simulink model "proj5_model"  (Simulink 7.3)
settings: Solver=FixedStepDiscrete  StartTime=0.0  StopTime=1.2  RelTol=1e-3
InitFcn:
  | clear
  | % Digital Modulation
  | M=4;                % MQAM
  | Fs=1e06;             % Symbols Rate
  | Fb=log2(M)*Fs;   % bit rate
  | 
  | % Power Transmitted and Received
  | PT=5.0;             % Transmitted Power in Watts
  | A=1/100;           % channel attenuation
  | PR=A*PT;          % Received Power in Watts
  | 
  | % channel
  | P=[0,-5, 5];   % dB
  | T=[0, 10 15]*10^(-6);  % sec
  | fd=60; %Hz
libraries: commrandsrc2 x1, commsink2 x1, commchan3 x1, commdigbbndam3 x1

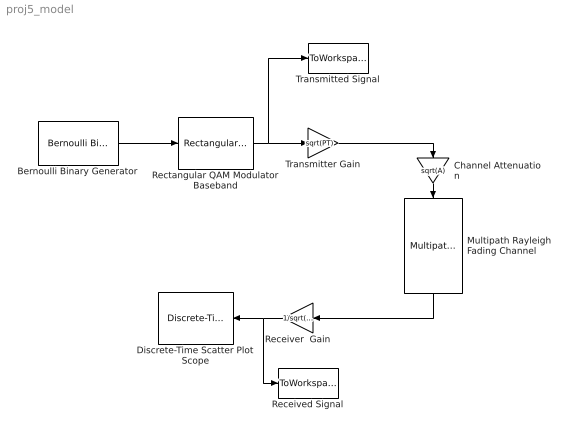
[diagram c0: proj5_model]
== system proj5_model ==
  Bernoulli Binary Generator : commrandsrc2/Bernoulli Binary Generator  DialogController=commDDGCreate  DialogControllerArgs=DataTag0  SystemSampleTime=-1  P=0.5  seed=61  Ts=1/Fb  frameBased=on  sampPerFrame=log2(M)*100  orient=off  outDataType=single
  Channel Attenuation : Gain  Gain=sqrt(A)  ParameterDataType=sfix(16)  ParameterScaling=2^0  OutDataType=sfix(16)  OutScaling=2^0
  Discrete-Time Scatter Plot Scope : commsink2/Discrete-Time Scatter Plot Scope  Tag=ScatterPlot  SystemSampleTime=-1  sampPerSymb=1  offsetEye=0  numTraces=40  numNewFrames=10  LineMarkers=.  LineColors=b  fading=on  render=on  AxisGrid=on  xMin=-3.3  xMax=3.315  yMin=-3.3  yMax=3.315  inphaseLabel=In-phase Amplitude  quadratureLabel=Quadrature Amplitude  openScopeAtSimStart=on  FrameNumber=off  FigPos=[232 106 560 560]  figTitle=Scatter Plot  numLinesMax=8  block_type_=scatter
  Multipath Rayleigh Fading Channel : commchan3/Multipath Rayleigh Fading Channel  SystemSampleTime=-1  maxDopplerShift=fd  spectrumType=Jakes  sigmaGaussian=1/sqrt(2)  coeffRounded=[1 -1.72 0.785]  freqMinMaxRJakes=[0 1]  freqMinMaxAJakes=[0 1]  sigmaGaussian1=1/sqrt(2)  sigmaGaussian2=1/sqrt(2)  centerFreqGaussian1=0.0  centerFreqGaussian2=0.0  gainGaussian1=0.5  gainGaussian2=0.5  coeffBell=9  dopplerSpectrum=doppler.jakes  pathDelays=T  avgPathGaindB=P  normalizePathGains=on  seed=73  enableProbe=0  openVisAtStart=off  outPathGains=off  outDelay=off
  Received Signal : ToWorkspace  VariableName=y  SampleTime=-1  SaveFormat=Array
  Receiver  Gain : Gain  Gain=1/sqrt(PR)  ParameterDataType=sfix(16)  ParameterScaling=2^0  OutDataType=sfix(16)  OutScaling=2^0
  Rectangular QAM Modulator Baseband : commdigbbndam3/Rectangular QAM Modulator Baseband  DialogController=commDDGCreate  DialogControllerArgs=DataTag1  M=M  InType=Bit  Enc=Gray  Mapping=[0:15]  PowType=Average Power  MinDist=2  AvgPow=1  PeakPow=1  Ph=0  outDtype=double  outWordLen=16  outUDDataType=sfix(16)  outFracLenMode=Best precision  outFracLen=15
  Transmitted Signal : ToWorkspace  VariableName=x  SampleTime=-1  SaveFormat=Array
  Transmitter Gain : Gain  Gain=sqrt(PT)  ParameterDataType=sfix(16)  ParameterScaling=2^0  OutDataType=sfix(16)  OutScaling=2^0
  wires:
  Bernoulli Binary Generator/1 -> Rectangular QAM Modulator Baseband/1
  Rectangular QAM Modulator Baseband/1 -> Transmitter Gain/1, Transmitted Signal/1
  Multipath Rayleigh Fading Channel/1 -> Receiver  Gain/1
  Transmitter Gain/1 -> Channel Attenuation/1
  Channel Attenuation/1 -> Multipath Rayleigh Fading Channel/1
  Receiver  Gain/1 -> Discrete-Time Scatter Plot Scope/1, Received Signal/1
